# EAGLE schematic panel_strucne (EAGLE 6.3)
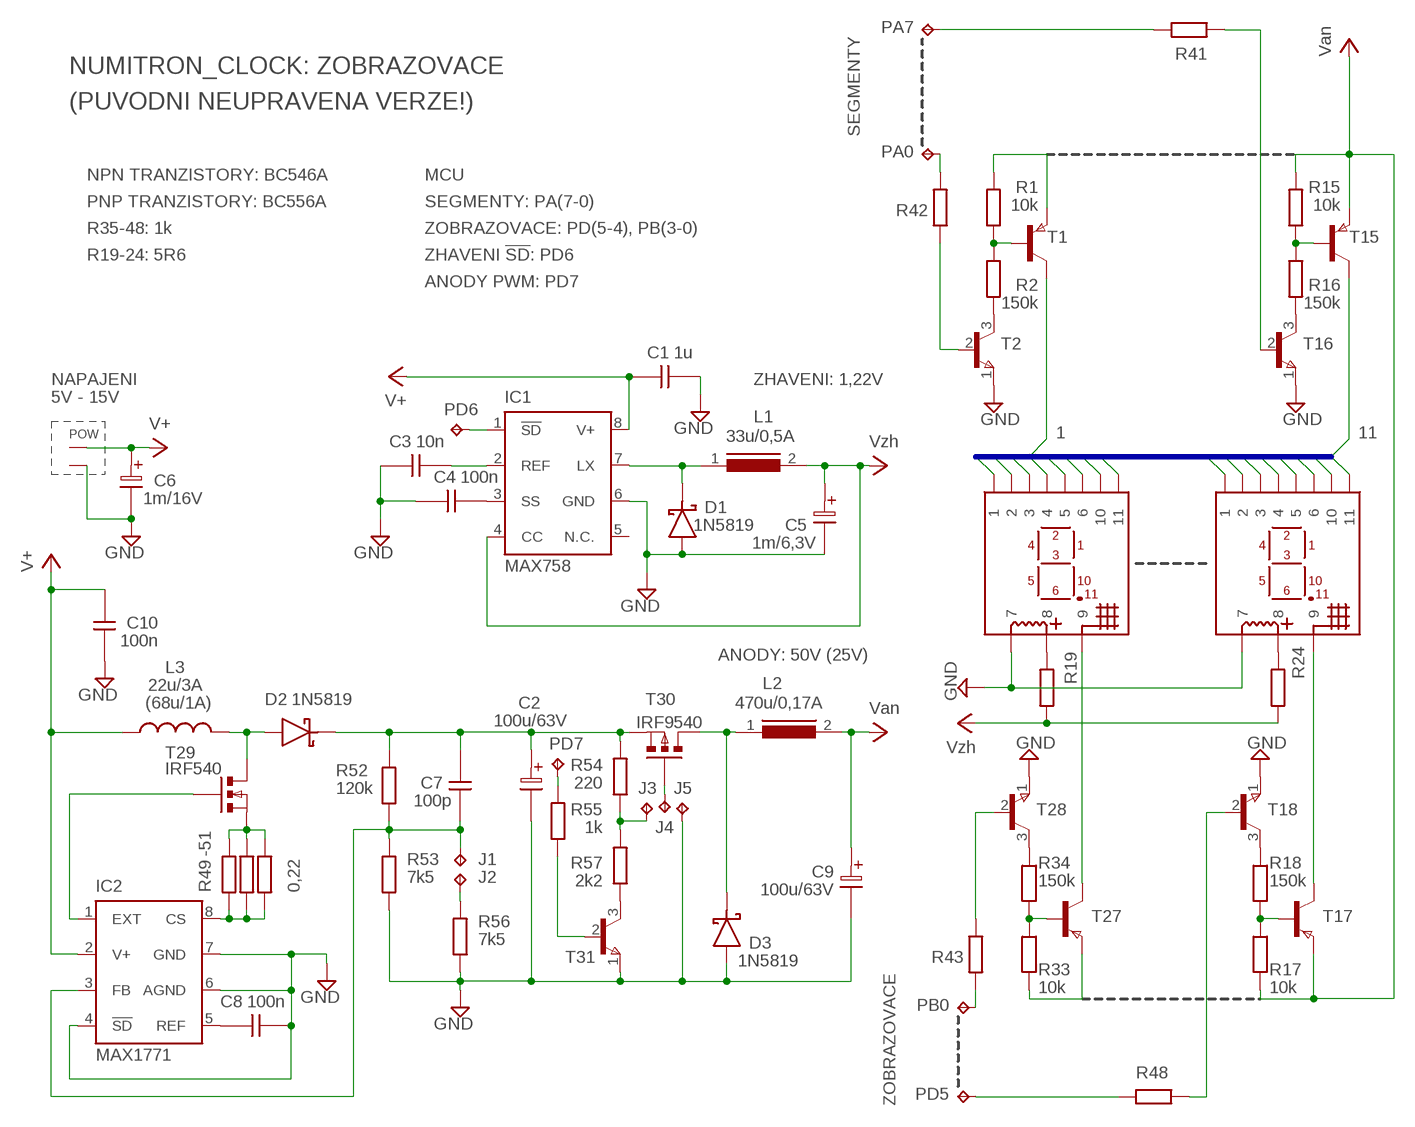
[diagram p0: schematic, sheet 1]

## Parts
C1  1u  CK  [CK]
C2  100u/63V  CT15  [CT15]
C3  10n  CK  [CK]
C4  100n  CK  [CK]
C5  1m/6,3V  CT15  [CT15]
C6  1m/16V  CT15  [CT15]
C7  100p  CK  [CK]
C8  100n  CK  [CK]
C9  100u/63V  CT15  [CT15]
C10  100n  CK  [CK]
D1  1N5819  [DO41]
D2  1N5819  [DO41]
D3  1N5819  [DO41]
IC1  MAX758  [DIL08]
IC2  MAX1771  [DIL08]
J1  TPPAD1-13Y  [P1-13Y]
J2  TPPAD1-13Y  [P1-13Y]
J3  TPPAD1-13Y  [P1-13Y]
J4  TPPAD1-13Y  [P1-13Y]
J5  TPPAD1-13Y  [P1-13Y]
L1  33u/0,5A  SMCC12  [SMCC12]
L2  470u/0,17A  SMCC12  [SMCC12]
L3  22u/3A  TOROID  [L_14X8]
PA0  TPPAD1-13Y  [P1-13Y]
PA7  TPPAD1-13Y  [P1-13Y]
PB0  TPPAD1-13Y  [P1-13Y]
PD5  TPPAD1-13Y  [P1-13Y]
PD6  TPPAD1-13Y  [P1-13Y]
PD7  TPPAD1-13Y  [P1-13Y]
POW  ARK500/2  [ARK500/2]
R1  10k  MRR  [MRR]
R2  150k  MRR  [MRR]
R15  10k  MRR  [MRR]
R16  150k  MRR  [MRR]
R17  10k  MRR  [MRR]
R18  150k  MRR  [MRR]
R19  MRR  [MRR]
R24  MRR  [MRR]
R33  10k  MRR  [MRR]
R34  150k  MRR  [MRR]
R41  MRR  [MRR]
R42  MRR  [MRR]
R43  MRR  [MRR]
R48  MRR  [MRR]
R49  0,22  MRR-10  [RR-10]
R50  0,22  MRR-10  [RR-10]
R51  0,22  MRR-10  [RR-10]
R52  120k  MRR  [MRR]
R53  7k5  MRR  [MRR]
R54  220  MRR  [MRR]
R55  1k  MRR  [MRR]
R56  7k5  MRR  [MRR]
R57  2k2  MRR  [MRR]
T1  BC556  BC556A  [TO-92C]
T2  BC546  BC546A  [TO-92C]
T15  BC546  BC556A  [TO-92C]
T16  BC546  BC546A  [TO-92C]
T17  BC546  BC556A  [TO-92C]
T18  BC546  BC546A  [TO-92C]
T27  BC546  BC556A  [TO-92C]
T28  BC546  BC546A  [TO-92C]
T29  IRF540  [D2PAK]
T30  IRF9540  [D2PAK]
T31  BC546  BC546A  [TO-92C]
U$1  IV6  [IV6]
U$6  IV6  [IV6]

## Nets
GND: C1.2 C2.2 C3.1 C4.1 C5.2 C6.2 C8.2 C9.2 C10.1 D1.A D3.A IC1.6(GND) IC2.4(!SD) IC2.6(AGND) IC2.7(GND) J5.TP POW.2 R53.2 R56.2 T2.1(E) T16.1(E) T18.1(E) T28.1(E) T31.1(E) U$1.P$7 U$6.P$7
N$1: R1.1 R2.2 T1.2(B)
N$2: R2.1 T2.3(C)
N$3: J2.TP R56.1
N$4: R1.2 T1.1(E)
N$6: PA0.TP R42.1
N$22: R15.1 R16.2 T15.2(B)
N$23: R16.1 T16.3(C)
N$25: R17.1 R18.2 T17.2(B)
N$26: R18.1 T18.3(C)
N$27: PA7.TP R41.2
N$28: R49.2 R50.2 R51.2 T29.S
N$29: R19.2 U$1.P$8
N$31: R33.2 T27.1(E)
N$34: R24.2 U$6.P$8
N$35: IC1.1(!SD) PD6.TP
N$48: R33.1 R34.2 T27.2(B)
N$49: R34.1 T28.3(C)
N$51: T17.3(C) U$6.P$9
N$56: T27.3(C) U$1.P$9
N$58: R42.2 T2.2(B)
N$59: R41.1 T16.2(B)
N$60: PB0.TP R43.2
N$61: R43.1 T28.2(B)
N$66: PD5.TP R48.1
N$67: R48.2 T18.2(B)
N$72: IC2.8(CS) R49.1 R50.1 R51.1
N$73: C4.2 IC1.3(SS)
N$74: D1.K IC1.7(LX) L1.1
N$75: C3.2 IC1.2(REF)
N$76: IC2.1(EXT) T29.G
N$77: R55.1 T31.2(B)
N$78: D2.A L3.P$4 T29.D
N$79: C7.1 IC2.3(FB) J1.TP R52.2 R53.1
N$80: C2.1 C7.2 D2.K R52.1 R54.2 T30.S
N$81: D3.K L2.1 T30.D
N$82: J4.TP T30.G
N$83: R57.1 T31.3(C)
N$84: PD7.TP R55.2
N$85: J3.TP R54.1 R57.2
N$87: C8.1 IC2.5(REF)
SEGMENTY0: T1.3(C) U$1.P$1 U$6.P$1
SEGMENTY1: U$1.P$2 U$6.P$2
SEGMENTY2: U$1.P$3 U$6.P$3
SEGMENTY3: U$1.P$4 U$6.P$4
SEGMENTY4: U$1.P$5 U$6.P$5
SEGMENTY5: U$1.P$6 U$6.P$6
SEGMENTY6: U$1.P$10 U$6.P$10
SEGMENTY7: T15.3(C) U$1.P$11 U$6.P$11
V+: C1.1 C6.1 IC1.8(V+) POW.1
VAN: C9.1 L2.2 R15.2 R17.2 T15.1(E) T17.1(E) ; supply symbol labelled Van
VCC: C10.2 IC2.2(V+) L3.P$3 ; supply symbol labelled V+
VZH: C5.1 IC1.4(CC) L1.2 R19.1 R24.1 ; supply symbol labelled Vzh
Unconnected: IC1.5(N.C.)

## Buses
SEGMENTY[0..7]

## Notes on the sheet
- NUMITRON_CLOCK: ZOBRAZOVACE
- (PUVODNI NEUPRAVENA VERZE!)
- SEGMENTY
- NPN TRANZISTORY: BC546A | MCU
- PNP TRANZISTORY: BC556A | SEGMENTY: PA(7-0)
- R35-48: 1k | ZOBRAZOVACE: PD(5-4), PB(3-0)
- R19-24: 5R6 | ZHAVENI !SD!: PD6
- ANODY PWM: PD7
- NAPAJENI | ZHAVENI: 1,22V
- 5V - 15V
- 1 | 11
- ANODY: 50V (25V)
- (68u/1A)
- -51
- ZOBRAZOVACE

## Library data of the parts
C1 C3 C4 C7 C8 C10 = #_GM99:CK
C2 C5 C6 C9 = #_GM99:CT15: RM = 5mm, R = 10mm
D1-D3 = #_GM99:1N5819
IC1 = #_my:MAX758
IC2 = #_my:MAX1771
J1-J5 PA0 PA7 PB0 PD5-PD7 = testpad:TP: Test pad
L1 L2 = inductors:SMCC12: INDUCTOR
L3 = #_my:TOROID
POW = #_GM99:ARK500/2
R1 R2 R15-R19 R24 R33 R34 R41-R43 R48 R52-R57 = #_GM99:MRR
R49-R51 = #_GM99:MRR-10
T1 T15 T17 T27 = #_GM99:BC556A
T2 T16 T18 T28 T31 = #_GM99:BC546A
T29 = #_my:IRF540
T30 = #_my:IRF9540
U$1 U$6 = #_my:IV6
